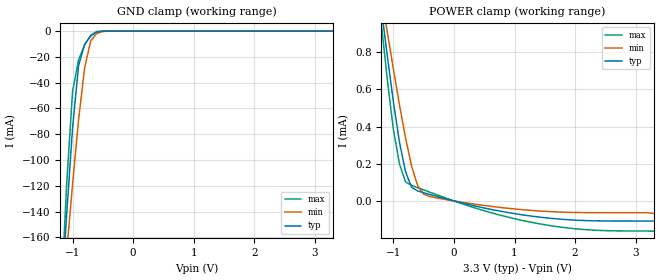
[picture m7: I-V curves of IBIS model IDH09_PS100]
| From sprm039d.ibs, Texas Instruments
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[Model]   IDH09_PS100
| Input with pullup
Model_type   Input
Polarity   Non-Inverting
| signals   A, Y
Vinl = 0.8V
Vinh = 2.0V
|   typ   min   max
C_comp   1.5797p   1.5046p   1.7659p
|   typ   min   max
[Temperature Range]   25   -40   125
|   typ   min   max
[Voltage Range]   3.30V   3.00V   3.60V
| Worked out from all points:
|   GND clamp passes 1 mA (typ) near -0.61 V on its own axis
|   POWER clamp passes 1 mA (typ) near -1.19 V on its own axis
[GND_clamp]
|   Voltage   I(typ)   I(min)   I(max)
-3.3V     -2.002A    -1.514A    -2.597A
-1.2V     -220.8mA   -229.8mA   -218.9mA
-1.1V     -144.4mA   -173.1mA   -120.7mA
-1V       -75.15mA   -118.7mA   -46.82mA
-900mV    -26.55mA   -68.65mA   -22.24mA
-800mV    -10.21mA   -28.33mA   -10.81mA
-700mV    -3.767mA   -7.526mA   -3.181mA
-600mV    -734.6uA   -1.835mA   -363.9uA
-500mV    -67.23uA   -328.9uA   -17.02uA
-400mV    -3.755uA   -40.45uA   -379.9nA
3.3V      177.6pA    34.37nA    -44.41pA
[POWER_clamp]
|   Voltage   I(typ)   I(min)   I(max)
-3.3V     6.839mA    5.575mA    7.991mA
-1.2V     1.035mA    1.107mA    953.9uA
-1.1V     776.9uA    904.7uA    648.7uA
-1V       531.1uA    707uA      381.7uA
-900mV    315.1uA    516.3uA    198.5uA
-800mV    157.1uA    338.5uA    102.2uA
-700mV    72.87uA    187.6uA    83.48uA
-600mV    53.6uA     82.48uA    71.35uA
-500mV    44.08uA    35.96uA    59.29uA
500mV     -38.01uA   -24.41uA   -52.73uA
1.4V      -86.4uA    -53.81uA   -122.3uA
3.3V      -108.3uA   -67.2uA    -162.1uA
